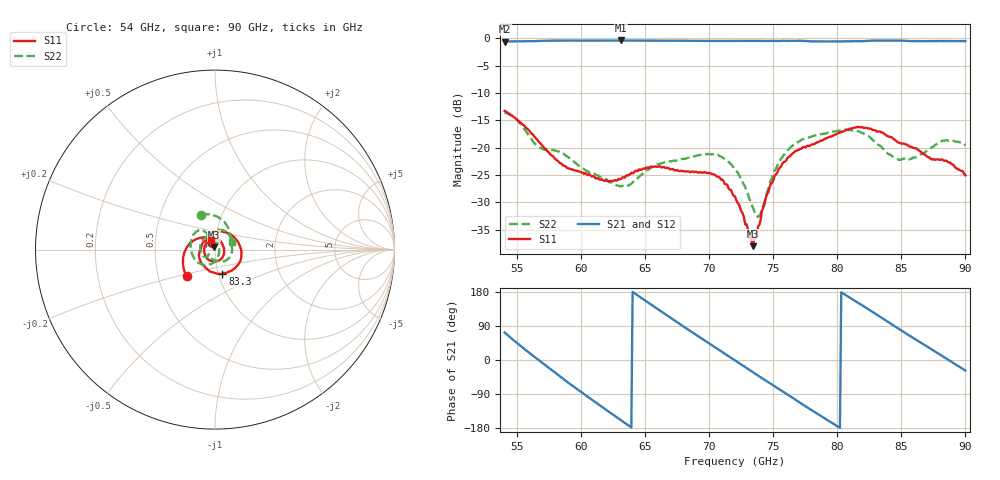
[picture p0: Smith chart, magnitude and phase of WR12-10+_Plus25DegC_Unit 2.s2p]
!Mini-Circuits Laboratory
!S-Parameters
!Model: WR12-10+
!Run / Lot / Date Code: Y97271 / QN2608234 / 2608
!Fixture: N/A, Pressing Arm: N/A
!Network Analyzer: PNA-X N5242B - 423 4 ports (COM/DCOM);  Serial number: 76642
!Date: 3/10/2026 at 2:21:43 PM
!No.: Unit# 2
!Tested with:
# Hz  S  dB  R  50
!Frequency  S11 dB  S11 Deg  S21 dB  S21 Deg  S12 dB  S12 Deg  S22 dB  S22 Deg
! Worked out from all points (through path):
!   352 points, 54 GHz to 90 GHz, reference 50 ohm
!   highest |S21| = -0.39 dB at 63.1 GHz (marker M1); lowest = -0.6 dB at 54 GHz (marker M2)
!   lowest |S11| = -38.0 dB at 73.4 GHz (marker M3), VSWR 1.03, Z = 49.6 + j1.19 ohm
!   |S11| at or under -10 dB: start of sweep to end of sweep
!   |S22| runs from -32.6 to -13.5 dB; largest |S21 - S12| = 0.044
!   S11 on the Smith chart (normalised r, x): 54 GHz: 0.70, -0.22; 83.3 GHz: 1.04, -0.29; 90 GHz: 0.96, +0.10
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5.4e10  -13.26 -136.8  -0.59 72.5  -0.55 73.7  -13.55 111.8
5.55e10  -15.92 177.5  -0.54 30.4  -0.51 31.3  -16.42 64.8
5.69e10  -19.45 142.2  -0.47 -6.5  -0.45 -5.6  -20.15 20.3
5.87e10  -23.32 107.2  -0.40 -52.9  -0.37 -52.0  -21.28 -43.4
6e10  -24.46 74.3  -0.42 -85.1  -0.39 -84.4  -23.64 -75.9
6.15e10  -25.84 38.6  -0.41 -121.0  -0.39 -120.8  -25.39 -113.6
6.31e10  -25.69 -11.0  -0.39 -159.2  -0.37 -159.0  -27.03 -144.2
6.45e10  -23.96 -59.7  -0.41 168.0  -0.39 168.0  -25.32 -138.0
6.6e10  -23.45 -112.3  -0.43 133.5  -0.41 133.4  -23.01 -146.6
6.87e10  -24.32 167.3  -0.46 72.3  -0.42 72.2  -21.62 174.7
7.04e10  -24.88 130.7  -0.48 34.4  -0.43 34.2  -21.27 133.8
7.2e10  -28.92 91.6  -0.47 -1.1  -0.45 -1.2  -23.89 97.0
7.34e10  -37.98 108.4  -0.46 -32.3  -0.45 -31.8  -30.92 42.9
7.39e10  -34.08 136.1  -0.46 -43.3  -0.46 -42.8  -32.51 -9.2
7.58e10  -22.62 121.1  -0.44 -84.5  -0.56 -84.4  -21.32 -107.4
7.8e10  -19.40 71.4  -0.56 -132.7  -0.54 -131.1  -17.94 -160.6
8.06e10  -16.82 2.4  -0.57 172.3  -0.56 172.9  -16.69 149.0
8.33e10  -17.01 -73.2  -0.42 114.6  -0.61 115.8  -19.57 116.2
8.4e10  -17.95 -96.5  -0.42 99.5  -0.58 101.0  -21.19 119.0
8.56e10  -19.71 -141.2  -0.50 65.0  -0.51 67.2  -22.16 116.6
8.74e10  -22.17 172.8  -0.49 27.3  -0.51 28.7  -19.88 95.3
9e10  -25.04 110.5  -0.51 -27.8  -0.45 -26.1  -19.58 22.6
